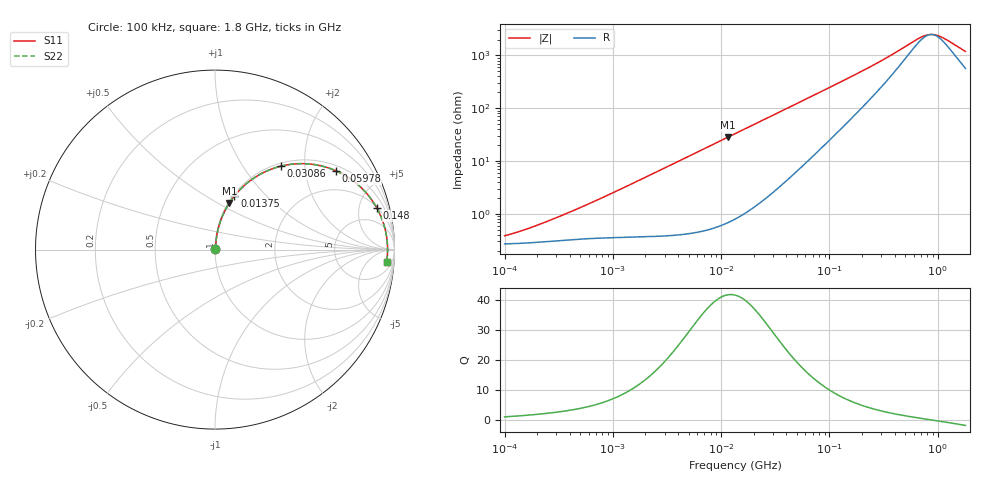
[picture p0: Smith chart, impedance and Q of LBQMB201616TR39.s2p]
! LBQMB201616TR39  S-PARAMETER MODEL  ( General Type )
! Model Generated by TAIYO YUDEN Corporation (http://www.ty-top.com)
! Version 1.0
! TAIYO YUDEN Control No. 191025NI43SB-FBB
! Copyright(c) 2019 TAIYO YUDEN CO.,LTD. All Rights Reserved.
! Product Description (link to TY-COMPAS)
! https://ds.yuden.co.jp/TYCOMPAS/or/detail?pn=LBQMB201616TR39J&u=M
! Products Name : Inductors
! Characteristics :
!  Inductance : 0.39 uH , SRF(min) : 375 MHz , DC Resistance(max) : 0.338 Ohm , Rated Current : 440 mA
!  Case Size : 2.0 x 1.6 / 0.079 x 0.063 [mm/inch] , Thickness : 1.6 / 0.063 [mm/inch]
!  (Conditions: Temperature = 25 degC , DC Bias Current/Voltage = 0A / 0V)
! External Node Assignments :
!  1  o---GGG---o  2
! GND o---------o GND
! Frequency Range : 0.1MHz  -  1800MHz  [ 402 STEP ]
# MHz S RI R 50
! Freq[MHz].  S11 Real  S11 Imag  S21 Real  S21 Imag  S12 Real  S12 Imag  S22 Real  S22 Imag
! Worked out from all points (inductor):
!   401 points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, 100 kHz to 1.8 GHz, reference 50 ohm
!   read as one part in series: L = 406 nH near 375.4 kHz
!   highest Q = 41.6 at 11.58 MHz (marker M1), where L = 390 nH
!   self-resonance near 873.2 MHz
!   S11 on the Smith chart (normalised r, x): 100 kHz: 1.01, +0.01; 13.75 MHz: 1.02, +0.67; 30.86 MHz: 1.05, +1.51; 59.78 MHz: 1.18, +2.93; 148 MHz: 2.10, +7.30; 1.8 GHz: 12, -21
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0.1  0.00269 0.00272  0.9973 -0.00272  0.9973 -0.00272  0.00269 0.00272
0.193745  0.00289 0.00516  0.9971 -0.00516  0.9971 -0.00516  0.00289 0.00516
0.516129  0.00349 0.013  0.9965 -0.013  0.9965 -0.013  0.00349 0.013
2.66389  0.00795 0.0646  0.992 -0.0646  0.992 -0.0646  0.00795 0.0646
5.833619  0.0242 0.1389  0.9758 -0.1389  0.9758 -0.1389  0.0242 0.1389
11.58263  0.0799 0.2594  0.9201 -0.2594  0.9201 -0.2594  0.0799 0.2594
13.41641  0.1033 0.2925  0.8967 -0.2925  0.8967 -0.2925  0.1033 0.2925
13.74911  0.1077 0.2982  0.8923 -0.2982  0.8923 -0.2982  0.1077 0.2982
20.3463  0.2056 0.3908  0.7944 -0.3908  0.7944 -0.3908  0.2056 0.3908
30.85563  0.3686 0.4652  0.6314 -0.4652  0.6314 -0.4652  0.3686 0.4652
42.42587  0.5193 0.4776  0.4807 -0.4776  0.4807 -0.4776  0.5193 0.4776
59.78129  0.6736 0.4392  0.3264 -0.4392  0.3264 -0.4392  0.6736 0.4392
69.24595  0.7297 0.4103  0.2703 -0.4103  0.2703 -0.4103  0.7297 0.4103
99.99243  0.8358 0.3234  0.1642 -0.3234  0.1642 -0.3234  0.8358 0.3234
147.9715  0.9015 0.2321  0.0985 -0.2321  0.0985 -0.2321  0.9015 0.2321
357.3983  0.9535 0.0871  0.0465 -0.0871  0.0465 -0.0871  0.9535 0.0871
659.3364  0.9609 0.0246  0.0391 -0.0246  0.0391 -0.0246  0.9609 0.0246
745.2431  0.9613 0.0137  0.0387 -0.0137  0.0387 -0.0137  0.9613 0.0137
842.3428  0.9615 0.0031  0.0385 -0.0031  0.0385 -0.0031  0.9615 0.0031
952.0939  0.9615 -0.00749  0.0385 0.00749  0.0385 0.00749  0.9615 -0.00749
1076.145  0.9612 -0.0182  0.0388 0.0182  0.0388 0.0182  0.9612 -0.0182
1800  0.9567 -0.0678  0.0433 0.0678  0.0433 0.0678  0.9567 -0.0678
